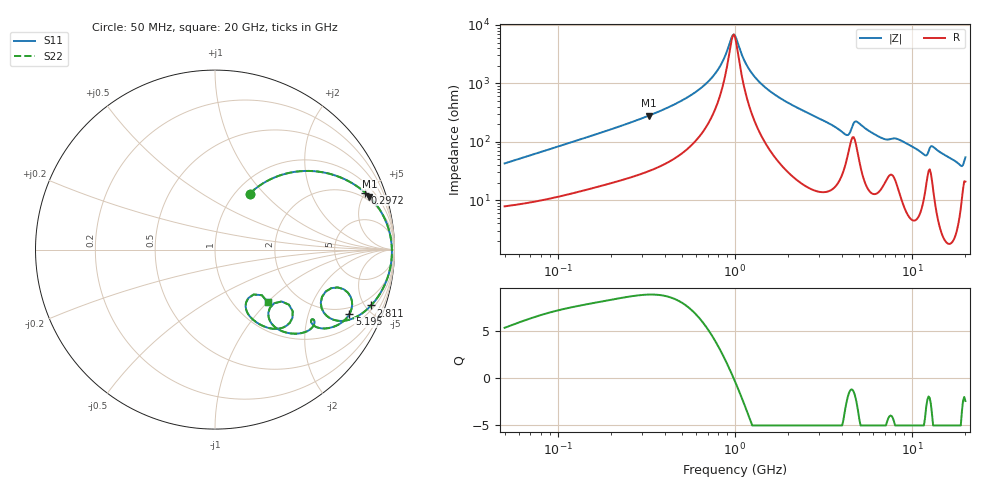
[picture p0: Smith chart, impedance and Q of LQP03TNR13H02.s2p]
!Murata Part Number: LQP03TNR13H02
!These Parameters are Measured in Series Mode Connection
!  o--[Z]--o
!Port1  Port2
!  o-------o
!Freq. Start=50[MHz] Stop=20[GHz], 401[Steps]
# Hz S RI R 50
!Freq.(Hz) S11(Real) S11(Imag) S21(Real) S21(Imag) S12(Real) S12(Imag) S22(Real) S22(Imag)
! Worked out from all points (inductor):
!   401 points, 50 MHz to 20 GHz, reference 50 ohm
!   read as one part in series: L = 131 nH near 51.52 MHz
!   highest Q = 8.86 at 325.2 MHz (marker M1), where L = 136 nH
!   self-resonance near 970.5 MHz
!   S11 on the Smith chart (normalised r, x): 50 MHz: 1.16, +0.84; 297.2 MHz: 1.57, +4.98; 2.811 GHz: 1.29, -5.47; 5.195 GHz: 1.61, -3.73; 20 GHz: 1.42, -1.00
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5e7  0.1936 0.3125  0.8064 -0.3125  0.8064 -0.3125  0.1936 0.3125
1.364002e8  0.5491 0.4371  0.4509 -0.4371  0.4509 -0.4371  0.5491 0.4371
2.972233e8  0.8367 0.3172  0.1633 -0.3172  0.1633 -0.3172  0.8367 0.3172
3.251725e8  0.8603 0.2948  0.1397 -0.2948  0.1397 -0.2948  0.8603 0.2948
3.721004e8  0.8912 0.2598  0.1088 -0.2598  0.1088 -0.2598  0.8912 0.2598
6.980337e8  0.9739 0.0905  0.0261 -0.0905  0.0261 -0.0905  0.9739 0.0905
8.108264e8  0.9815 0.0508  0.0185 -0.0508  0.0185 -0.0508  0.9815 0.0508
9.560587e8  0.9854 0.0072  0.0146 -0.0072  0.0146 -0.0072  0.9854 0.0072
1e9  0.9857 -0.00473  0.0143 0.00473  0.0143 0.00473  0.9857 -0.00473
1.161586e9  0.9845 -0.0449  0.0155 0.0449  0.0155 0.0449  0.9845 -0.0449
1.390315e9  0.9779 -0.0942  0.0221 0.0942  0.0221 0.0942  0.9779 -0.0942
2.728004e9  0.8788 -0.3009  0.1212 0.3009  0.1212 0.3009  0.8788 -0.3009
2.810964e9  0.8698 -0.3108  0.1302 0.3108  0.1302 0.3108  0.8698 -0.3108
4.275624e9  0.594 -0.3268  0.406 0.3268  0.406 0.3268  0.594 -0.3268
4.608136e9  0.6833 -0.2106  0.3167 0.2106  0.3167 0.2106  0.6833 -0.2106
5.194772e9  0.7484 -0.3602  0.2516 0.3602  0.2516 0.3602  0.7484 -0.3602
7.442007e9  0.5377 -0.39  0.4623 0.39  0.4623 0.39  0.5377 -0.39
1.004137e10  0.4089 -0.4648  0.5911 0.4648  0.5911 0.4648  0.4089 -0.4648
1.238412e10  0.371 -0.289  0.629 0.289  0.629 0.289  0.371 -0.289
1.438523e10  0.3138 -0.4398  0.6862 0.4398  0.6862 0.4398  0.3138 -0.4398
1.828096e10  0.1734 -0.3336  0.8266 0.3336  0.8266 0.3336  0.1734 -0.3336
2e10  0.2931 -0.2926  0.7069 0.2926  0.7069 0.2926  0.2931 -0.2926
